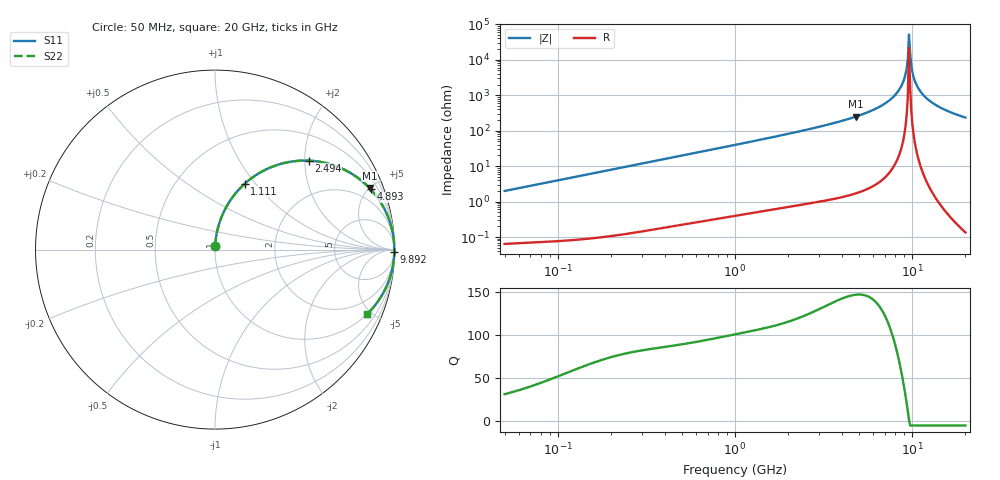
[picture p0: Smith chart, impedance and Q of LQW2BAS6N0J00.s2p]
!Murata Part Number: LQW2BAS6N0J00
!These Parameters are Measured in Series Mode Connection
!  o--[Z]--o
!Port1  Port2
!  o-------o
!Freq. Start=50[MHz] Stop=20[GHz], 401[Steps]
# Hz S RI R 50
!Freq.(Hz) S11(Real) S11(Imag) S21(Real) S21(Imag) S12(Real) S12(Imag) S22(Real) S22(Imag)
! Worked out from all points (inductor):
!   401 points, 50 MHz to 20 GHz, reference 50 ohm
!   read as one part in series: L = 6.35 nH near 51.52 MHz
!   highest Q = 147 at 4.82 GHz (marker M1), where L = 8.27 nH
!   self-resonance near 9.6 GHz
!   S11 on the Smith chart (normalised r, x): 50 MHz: 1.00, +0.04; 1.111 GHz: 1.01, +0.88; 2.494 GHz: 1.02, +2.09; 4.893 GHz: 1.04, +5.14; 9.892 GHz: open; 20 GHz: 1.00, -4.70
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5e7  0.00104 0.02  0.999 -0.02  0.999 -0.02  0.00104 0.02
1.364002e8  0.00378 0.0539  0.9962 -0.0539  0.9962 -0.0539  0.00378 0.0539
3.721004e8  0.0229 0.1437  0.9771 -0.1437  0.9771 -0.1437  0.0229 0.1437
1e9  0.1387 0.3407  0.8613 -0.3407  0.8613 -0.3407  0.1387 0.3407
1.110545e9  0.1657 0.367  0.8343 -0.367  0.8343 -0.367  0.1657 0.367
2.493527e9  0.5214 0.4955  0.4786 -0.4955  0.4786 -0.4955  0.5214 0.4955
2.728004e9  0.5723 0.4908  0.4277 -0.4908  0.4277 -0.4908  0.5723 0.4908
4.81993e9  0.8609 0.3427  0.1391 -0.3427  0.1391 -0.3427  0.8609 0.3427
4.89267e9  0.8667 0.3365  0.1333 -0.3365  0.1333 -0.3365  0.8667 0.3365
7.442007e9  0.9798 0.1361  0.0202 -0.1361  0.0202 -0.1361  0.9798 0.1361
8.141811e9  0.9909 0.0892  0.0091 -0.0892  0.0091 -0.0892  0.9909 0.0892
8.774992e9  0.9966 0.0496  0.0034 -0.0496  0.0034 -0.0496  0.9966 0.0496
9.178299e9  0.9985 0.0257  0.00153 -0.0257  0.00153 -0.0257  0.9985 0.0257
9.316812e9  0.9988 0.0177  0.00116 -0.0177  0.00116 -0.0177  0.9988 0.0177
9.457416e9  0.9991 0.00973  0.000918 -0.00973  0.000918 -0.00973  0.9991 0.00973
9.745021e9  0.9992 -0.00623  0.00082 0.00623  0.00082 0.00623  0.9992 -0.00623
9.892087e9  0.999 -0.0142  0.000963 0.0142  0.000963 0.0142  0.999 -0.0142
1.004137e10  0.9988 -0.0222  0.00123 0.0222  0.00123 0.0222  0.9988 -0.0222
1.034674e10  0.9978 -0.0381  0.00216 0.0381  0.00216 0.0381  0.9978 -0.0381
1.166392e10  0.989 -0.1016  0.011 0.1016  0.011 0.1016  0.989 -0.1016
1.438523e10  0.9535 -0.2096  0.0465 0.2096  0.0465 0.2096  0.9535 -0.2096
2e10  0.8465 -0.3602  0.1535 0.3602  0.1535 0.3602  0.8465 -0.3602
